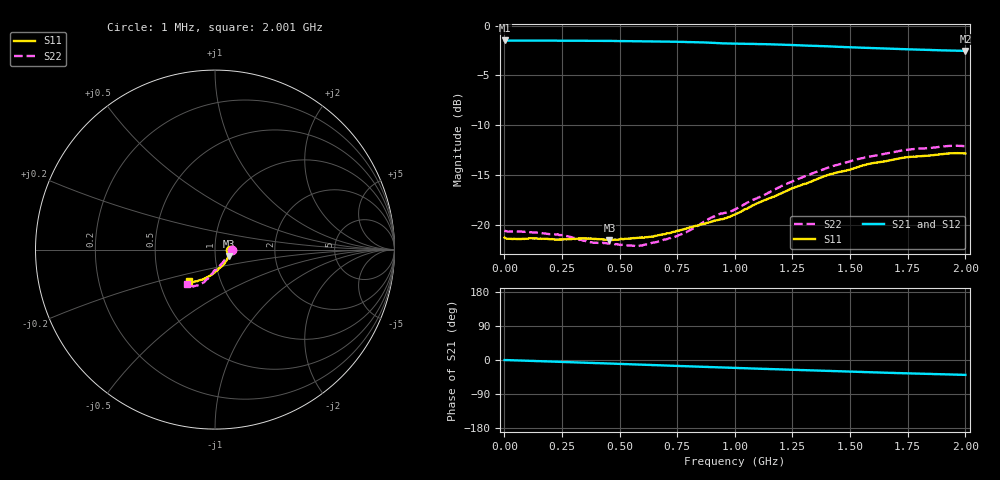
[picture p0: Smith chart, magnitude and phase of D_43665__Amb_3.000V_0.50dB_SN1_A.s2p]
! device id: 43665_
! dir: \\malibu\benchdata\1_engineers\tn_data\43665_75ohm\new\sparar\43665_\amb\3p000v\0p50db
! Serial: 1
! Insertion: A
! Temp: Amb
! VDD: 3.000V
! Attenuation Step: 0.50dB
! IDD: 1.453882e+00mA
! FILE NAME
! DATE 03-27-2009 08:33:29
! CORRECTED  DATA
#  Hz  S  RI  R  75
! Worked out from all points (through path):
!   401 points, 1 MHz to 2.001 GHz, reference 75 ohm
!   highest |S21| = -1.50 dB at 1 MHz (marker M1); lowest = -2.5 dB at 2.001 GHz (marker M2)
!   group delay of S21, straight-line fit = 55.8 ps
!   lowest |S11| = -21.5 dB at 456 MHz (marker M3), VSWR 1.18, Z = 87.1 - j6.11 ohm
!   |S11| at or under -10 dB: start of sweep to end of sweep
!   |S22| runs from -22.2 to -12.1 dB; largest |S21 - S12| = 0.0049
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1000000  0.0859 -0.00125  0.8417 -0.00133  0.8419 -0.00132  0.0934 -0.00132
2.26e8  0.0829 -0.0142  0.837 -0.0666  0.8372 -0.0669  0.0875 -0.0173
3.36e8  0.0819 -0.0236  0.8326 -0.0995  0.8328 -0.0998  0.0795 -0.0256
3.86e8  0.0803 -0.0281  0.8301 -0.114  0.8301 -0.1145  0.0749 -0.0309
4.56e8  0.0761 -0.0348  0.8261 -0.1353  0.8261 -0.1359  0.0703 -0.0396
5.76e8  0.0695 -0.0501  0.816 -0.1712  0.8159 -0.1716  0.0564 -0.0546
6.71e8  0.0615 -0.0636  0.8075 -0.1992  0.8072 -0.1995  0.0459 -0.0684
7.61e8  0.0521 -0.0778  0.7969 -0.2262  0.7969 -0.2264  0.0341 -0.082
8.01e8  0.0472 -0.0843  0.7915 -0.2383  0.7914 -0.2384  0.0276 -0.089
9.16e8  0.0267 -0.1013  0.7712 -0.2709  0.7716 -0.2707  0.00953 -0.1104
9.56e8  0.0218 -0.1052  0.7641 -0.2786  0.7645 -0.2784  0.000311 -0.1145
1.001e9  0.0166 -0.1112  0.7593 -0.2884  0.7599 -0.2884  -0.00599 -0.119
1.096e9  -0.00239 -0.1276  0.7449 -0.3132  0.7457 -0.3136  -0.0166 -0.1345
1.211e9  -0.0243 -0.1432  0.725 -0.3421  0.726 -0.3431  -0.0326 -0.1543
1.336e9  -0.0504 -0.1575  0.7003 -0.3682  0.7014 -0.3694  -0.053 -0.1728
1.406e9  -0.0654 -0.1654  0.6862 -0.3833  0.6872 -0.3853  -0.0627 -0.1831
1.521e9  -0.0877 -0.1713  0.6639 -0.4026  0.6641 -0.4052  -0.0841 -0.1939
1.581e9  -0.0987 -0.1762  0.6523 -0.4131  0.6522 -0.4163  -0.0926 -0.1982
1.671e9  -0.1123 -0.1776  0.6354 -0.4269  0.634 -0.4297  -0.1085 -0.2018
1.791e9  -0.1273 -0.1794  0.6135 -0.444  0.6109 -0.4475  -0.1266 -0.2045
1.931e9  -0.141 -0.1791  0.5889 -0.4629  0.5868 -0.4638  -0.1489 -0.1988
2.001e9  -0.1439 -0.1764  0.5773 -0.4723  0.5727 -0.4739  -0.1567 -0.1923
